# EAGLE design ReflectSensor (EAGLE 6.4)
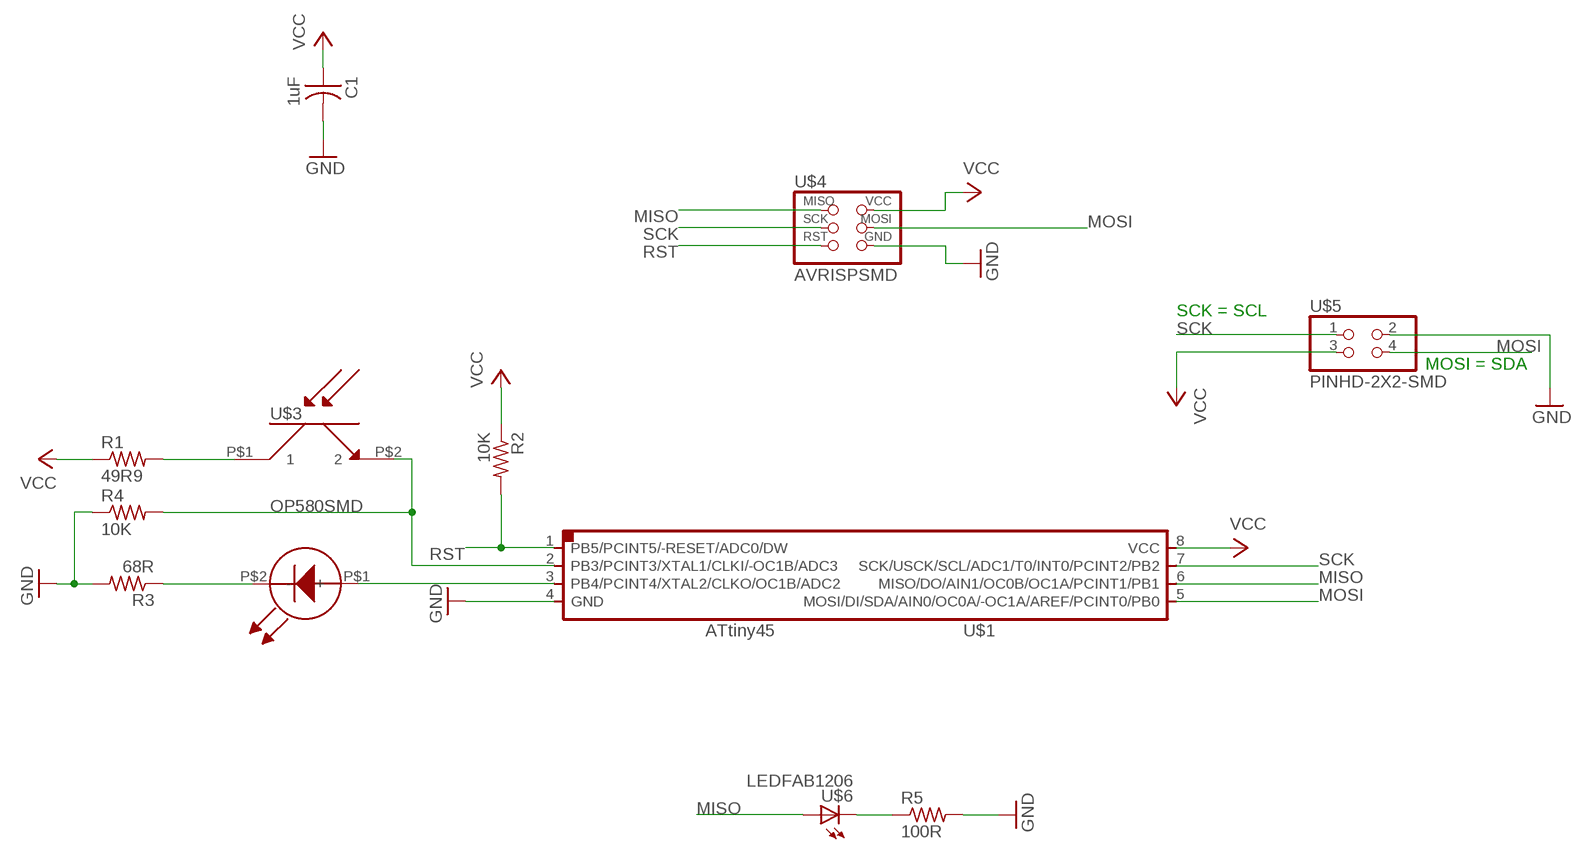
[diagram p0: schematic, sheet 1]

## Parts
C1  1uF  CAP-US1206FAB  [C1206FAB]
R1  49R9  RES-US1206FAB  [R1206FAB]
R2  10K  RES-US1206FAB  [R1206FAB]
R3  68R  RES-US1206FAB  [R1206FAB]
R4  10K  RES-US1206FAB  [R1206FAB]
R5  100R  RES-US1206FAB  [R1206FAB]
U$1  ATTINY45SI  [SOIC8]
U$2  OP280SMD  [OP280]
U$3  OP580SMD  [OP580]
U$4  AVRISPSMD  [2X03SMD]
U$5  PINHD-2X2-SMD  [2X02SMD]
U$6  LEDFAB1206  [LED1206FAB]

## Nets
GND: C1.2 R3.2 R4.1 R5.2 U$1.4(GND) U$4.6(GND) U$5.2
MISO: U$1.6(MISO/DO/AIN1/OC0B/OC1A/PCINT1/PB1) U$4.1(MISO) U$6.1(A)
MOSI: U$1.5(MOSI/DI/SDA/AIN0/OC0A/-OC1A/AREF/PCINT0/PB0) U$4.4(MOSI) U$5.4
N$1: R4.2 U$1.2(PB3/PCINT3/XTAL1/CLKI/-OC1B/ADC3) U$3.P$2
N$2: R1.2 U$3.P$1
N$3: U$1.3(PB4/PCINT4/XTAL2/CLKO/OC1B/ADC2) U$2.P$1(+)
N$4: R3.1 U$2.P$2(-)
N$5: R5.1 U$6.2(C)
RST: R2.2 U$1.1(PB5/PCINT5/-RESET/ADC0/DW) U$4.5(RST)
SCK: U$1.7(SCK/USCK/SCL/ADC1/T0/INT0/PCINT2/PB2) U$4.3(SCK) U$5.1
VCC: C1.1 R1.1 R2.1 U$1.8(VCC) U$4.2(VCC) U$5.3

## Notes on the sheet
- SCK = SCL
- MOSI = SDA

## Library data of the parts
C1 = fab:CAP-US
R1-R5 = fab:RES-US: Resistor (US Symbol)
U$1 = fab:ATTINY45
U$2 = Optics:OP280
U$3 = Optics:OP580
U$4 = fab:AVRISP
U$5 = fab:PINHD-2X2-SMD
U$6 = fab:LED: LED

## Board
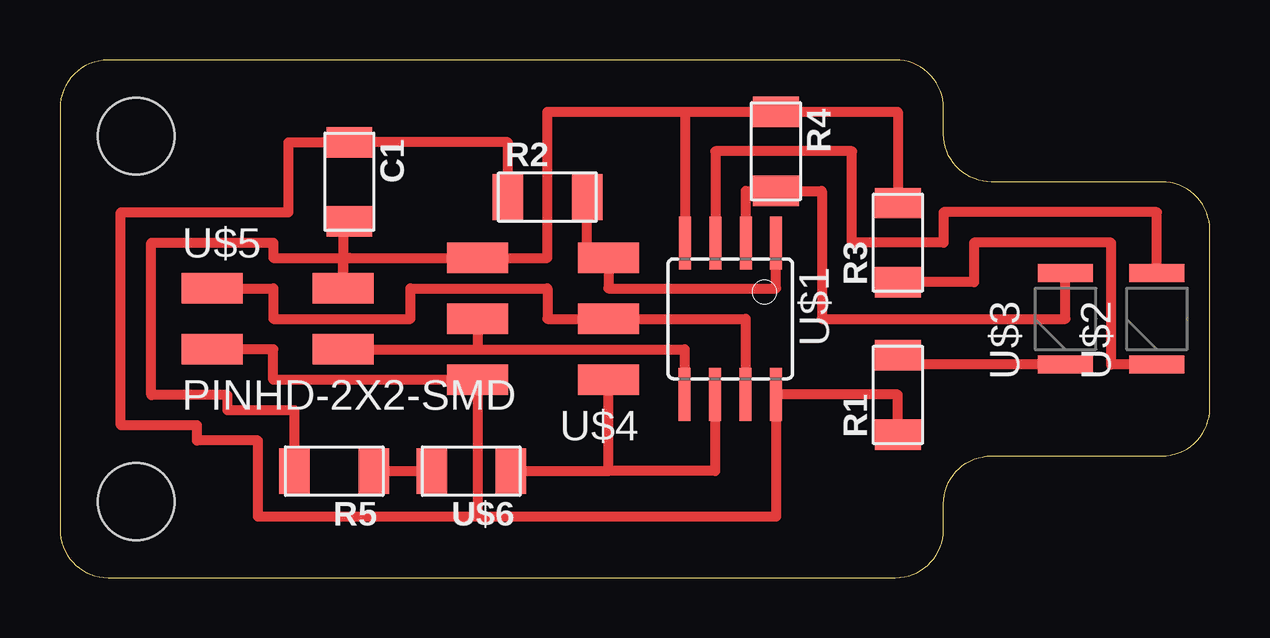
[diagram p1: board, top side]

Size 47.93 x 21.59 mm. Coordinates in mm from the lower left corner, seen from the top.
Outline: 36.83,18.5 36.83,19.59 arc90 34.83,21.59 2,21.58 arc90 0,19.58 0,2 arc90 2,0 34.83,0 arc90 36.83,2 36.83,3.08 arc-90 38.83,5.08 45.93,5.08 arc90 47.93,7.08 47.93,14.5 arc90 45.93,16.5 38.83,16.5 arc-90 36.83,18.5
Copper layers (1*16): Top 0.035mm / dielectric 1.5mm / Bottom 0.035mm
Design rules "fabmodule": minimum track width 10mil, minimum drill 0.4mm, track to track 0.42mm, track to pad 0.42mm, pad to pad 0.42mm, via to via 0.42mm, smd to smd 0.42mm, copper to edge 40mil, drill to drill 0.8mm, minimum pad ring 10mil, minimum via ring 8mil, stop-mask expansion 4mil, vias tented up to drill 0mil, thermal gap 10mil
Holes 3.2 mm at 3.17,18.41 3.17,3.17

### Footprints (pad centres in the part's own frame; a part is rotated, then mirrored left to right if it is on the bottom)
C1206FAB = smd 1.27 x 1.905: 1 -1.651,0; 2 1.651,0
R1206FAB = smd 1.27 x 1.905: 1 -1.651,0; 2 1.651,0
SOIC8 = smd 0.5 x 2.2: 1 -1.905,-3.154; 2 -0.645,-3.154; 3 0.625,-3.154; 4 1.895,-3.154; 5 1.905,3.154; 6 0.635,3.154; 7 -0.635,3.154; 8 -1.905,3.154
OP280 = smd 0.762 x 2.286: P$1 1.905,0; P$2 -1.905,0
OP580 = smd 0.762 x 2.286: P$1 -1.905,0; P$2 1.905,0
2X03SMD = smd 2.54 x 1.27: 1 -2.54,2.54; 2 2.92,2.54; 3 -2.54,0; 4 2.92,0; 5 -2.54,-2.54; 6 2.92,-2.54
2X02SMD = smd 2.54 x 1.27: 1 -2.54,1.27; 2 2.92,1.27; 3 -2.54,-1.27; 4 2.92,-1.27
LED1206FAB = smd 1.27 x 1.905: 1 -1.651,0; 2 1.651,0

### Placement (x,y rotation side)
C1  12.06,16.51 270 top
R1  34.92,7.62 90 top
R2  20.32,15.88 0 top
R3  34.92,13.97 90 top
R4  29.84,17.78 270 top
R5  11.43,4.45 180 top
U$1  27.94,10.79 180 top
U$2  45.72,10.79 90 top
U$3  41.91,10.79 90 top
U$4  20.32,10.79 180 top
U$5  8.89,10.79 0 top
U$6  17.14,4.45 180 top

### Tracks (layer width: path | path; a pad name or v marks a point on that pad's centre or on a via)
GND
  Top 0.406: 11.81,13.34 U$5.2 11.81,14.6 arc-90 C1.2 | 11.81,13.34 12.06,13.34 U$4.6 20.32,13.34 20.32,19.43 26.05,19.43 | 26.05,19.43 U$1.4 | 26.05,19.43 R4.1 34.92,19.43 R3.2 | R5.2 9.78,6.99 6.99,6.99 6.99,7.62 3.81,7.62 3.81,13.97 8.89,13.97 8.89,13.34 11.81,13.34
MISO
  Top 0.406: U$6.1 22.86,4.45 | 22.86,4.45 U$4.1 | U$1.6 27.3,4.45 22.86,4.45
MOSI
  Top 0.406: U$5.4 17.4,9.53 | U$4.4 17.4,9.53 | 17.4,9.53 26.04,9.53 U$1.5
N$1
  Top 0.406: U$1.2 28.59,16.13 R4.2 31.75,16.13 31.75,10.79 41.91,10.79 U$3.P$2
N$2
  Top 0.406: U$3.P$1 34.92,8.89 R1.2
N$3
  Top 0.406: U$2.P$1 45.72,15.24 36.83,15.24 36.83,13.97 33.02,13.97 33.02,17.78 27.32,17.78 | 27.3,17.78 27.32,17.78 | 27.32,17.78 U$1.3
N$4
  Top 0.406: U$2.P$2 43.81,8.89 43.81,13.97 38.1,13.97 38.1,12.32 R3.1
N$5
  Top 0.406: R5.1 U$6.2
RST
  Top 0.406: U$1.1 29.84,12.06 22.86,12.06 U$4.5 21.97,13.34 R2.2
SCK
  Top 0.406: U$5.1 8.89,12.06 8.89,10.79 14.61,10.79 14.61,12.06 20.32,12.06 20.32,10.79 U$4.3 28.57,10.79 U$1.7
VCC
  Top 0.406: R2.1 18.67,18.16 C1.1 9.53,18.16 9.53,15.24 2.54,15.24 2.54,6.35 5.71,6.35 5.71,5.71 8.26,5.71 8.26,2.54 17.4,2.54 | U$5.3 8.89,9.53 8.89,8.26 U$4.2 17.4,2.54 | R1.1 34.92,7.64 U$1.8 29.84,2.54 17.4,2.54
